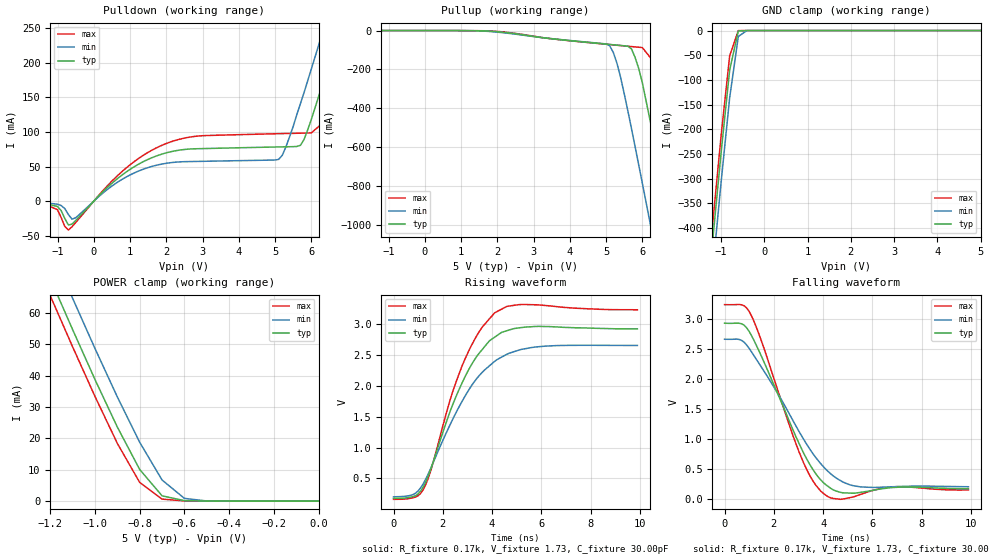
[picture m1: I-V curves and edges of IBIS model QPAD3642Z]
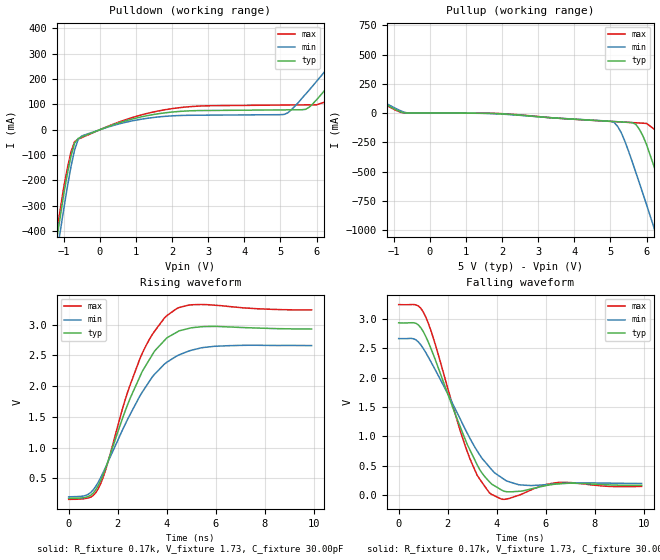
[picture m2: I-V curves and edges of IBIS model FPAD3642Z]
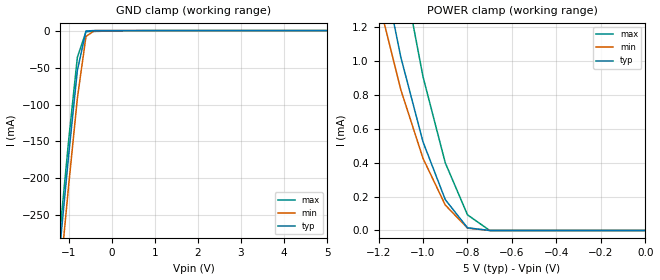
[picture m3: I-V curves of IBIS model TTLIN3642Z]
| IBIS file 723646.ibs created by s2ibis2 version 1.1
| North Carolina State University Electronics Research Laboratory  1995
[IBIS ver]   2.1
[File name]   723646.ibs
[File Rev]   1.0
[Date]   08/22/97
[Source]   Integrated Device Technology, Inc.
[Notes]   1. Temperatures: typ=25C, min=70C, max=0C 2. Cemos7_5v
   process. 3. Ramp rates based on 50 ohm load.
[Copyright]   Copyright 1997, Integrated Device Technology, Inc.
|   Component idt723646
[Component]   idt723646
[Manufacturer]   Integrated Device Technology
[Package]
| variable   typ   min   max
R_pkg   0.75   0.60   0.90
L_pkg   8.10nH   8.30nH   9.90nH
C_pkg   0.53pF   0.46pF   0.60pF
[Pin]  signal_name   model_name   R_pin   L_pin   C_pin
1   W_RA   TTLIN3642Z
2   ENA   TTLIN3642Z
3   CLKA   TTLIN3642Z
4   GND   GND
5   A35   QPAD3642Z
6   A34   QPAD3642Z
7   A33   QPAD3642Z
8   A32   QPAD3642Z
9   VCC   POWER
10   A31   QPAD3642Z
11   A30   QPAD3642Z
12   GND   GND
13   A29   QPAD3642Z
14   A28   QPAD3642Z
15   A27   QPAD3642Z
16   A26   QPAD3642Z
17   A25   QPAD3642Z
18   A24   QPAD3642Z
19   A23   QPAD3642Z
20   BEFWFTL   TTLIN3642Z
21   GND   GND
22   A22   QPAD3642Z
23   VCC   POWER
24   A21   QPAD3642Z
25   A20   QPAD3642Z
26   A19   QPAD3642Z
27   A18   QPAD3642Z
28   GND   GND
29   A17   QPAD3642Z
30   A16   QPAD3642Z
31   A15   QPAD3642Z
32   A14   QPAD3642Z
33   A13   QPAD3642Z
34   VCC   POWER
35   A12   QPAD3642Z
36   GND   GND
37   A11   QPAD3642Z
38   A10   QPAD3642Z
39   A9   QPAD3642Z
40   A8   QPAD3642Z
41   A7   QPAD3642Z
42   A6   QPAD3642Z
43   GND   GND
44   A5   QPAD3642Z
45   A4   QPAD3642Z
46   A3   QPAD3642Z
47   SPML   TTLIN3642Z
48   VCC   POWER
49   A2   QPAD3642Z
50   A1   QPAD3642Z
51   A0   QPAD3642Z
52   GND   GND
53   B0   QPAD3642Z
54   B1   QPAD3642Z
55   B2   QPAD3642Z
56   B3   QPAD3642Z
57   B4   QPAD3642Z
58   B5   QPAD3642Z
59   GND   GND
60   B6   QPAD3642Z
61   VCC   POWER
62   B7   QPAD3642Z
63   B8   QPAD3642Z
64   B9   QPAD3642Z
65   B10   QPAD3642Z
66   B11   QPAD3642Z
67   GND   GND
68   B12   QPAD3642Z
69   B13   QPAD3642Z
70   B14   QPAD3642Z
71   B15   QPAD3642Z
72   VCC   POWER
73   SIZEC   TTLIN3642Z
74   B16   QPAD3642Z
75   B17   QPAD3642Z
76   GND   GND
77   C0   QPAD3642Z
78   C1   QPAD3642Z
79   C2   QPAD3642Z
80   C3   QPAD3642Z
81   C4   QPAD3642Z
82   C5   QPAD3642Z
83   GND   GND
84   SIZEB   TTLIN3642Z
85   C6   QPAD3642Z
86   C7   QPAD3642Z
87   VCC   POWER
88   C8   QPAD3642Z
89   C9   QPAD3642Z
90   C10   QPAD3642Z
91   C11   QPAD3642Z
92   C12   QPAD3642Z
93   C13   QPAD3642Z
94   MBC   TTLIN3642Z
95   GND   GND
96   C14   QPAD3642Z
97   C15   QPAD3642Z
98   C16   QPAD3642Z
99   C17   QPAD3642Z
100   VCC   POWER
101   PRS2L   TTLIN3642Z
102   CLKB   TTLIN3642Z
103   ENB   TTLIN3642Z
104   W_RB   TTLIN3642Z
105   CSBL   TTLIN3642Z
106   GND   GND
107   FFCLIR   FPAD3642Z
108   EFBLOR   FPAD3642Z
109   AFCL   FPAD3642Z
110   AEBL   FPAD3642Z
111   VCC   POWER
112   MBF1   FPAD3642Z
113   MBB   TTLIN3642Z
114   MRS2L   TTLIN3642Z
115   FS1   TTLIN3642Z
116   GND   GND
117   CLKC   TTLIN3642Z
118   FS0   TTLIN3642Z
119   MRS1L   TTLIN3642Z
120   MBA   TTLIN3642Z
121   MBF2   FPAD3642Z
122   AEAL   FPAD3642Z
123   AFAL   FPAD3642Z
124   VCC   POWER
125   PRS1L   TTLIN3642Z
126   EFALOR   FPAD3642Z
127   FFALIR   FPAD3642Z
128   CSAL   TTLIN3642Z
| Models and submodels in the file (3): QPAD3642Z (I/O), FPAD3642Z (Output), TTLIN3642Z (Input)
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| FIN  FIN   dummy_model
| QIN  QIN   dummy_model
| QOEL QOEL   dummy_model
|   Model QPAD3642Z
[Model]   QPAD3642Z
Model_type   I/O
Polarity   Non-Inverting
Enable   Active-Low
Vinl =  0.000V
Vinh =  3.000V
Vmeas =  1.500V
C_comp   3.00pF   NA   NA
[Temperature Range]   25.00   70.00   0.000
[Voltage Range]   5.00V   4.50V   5.50V
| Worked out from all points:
|   slope of the pulldown table from 0 to 0.75 V, typ, clamps not added: 20.5 ohm
|   slope of the pullup table from 0 to 0.75 V, typ, clamps not added: 25.9 kohm
|   GND clamp passes 1 mA (typ) near -0.60 V on its own axis
|   POWER clamp passes 1 mA (typ) near -0.66 V on its own axis
|   rising waveform, R_fixture 0.17k, V_fixture 1.73, C_fixture 30.00pF: 20-80 % time 1.64ns typ, 1.93ns min, 1.5ns max; typ from 0.176 V to 2.93 V
|   falling waveform, R_fixture 0.17k, V_fixture 1.73, C_fixture 30.00pF: 20-80 % time 1.77ns typ, 2.16ns min, 1.53ns max; typ from 2.93 V to 0.173 V
[Pulldown]
| voltage   I(typ)   I(min)   I(max)
-5V       0A         -1mA       0A
-1.4V     -2.6mA     -1.9mA     -3.1mA
-1V       -7.7mA     -4.4mA     -12.4mA
-700mV    -34.39mA   -19.37mA   -41.73mA
700mV     34.57mA    28.94mA    39.05mA
1.8V      66.7mA     52.82mA    78.9mA
5.1V      78.42mA    60.43mA    97.58mA
5.7V      80.72mA    141mA      98.3mA
6.4V      184mA      259mA      117mA
6.8V      252mA      327mA      181mA
7.2V      320mA      396mA      249mA
10V       806mA      882mA      734mA
[Pullup]
| voltage   I(typ)   I(min)   I(max)
-5V       0A         0A         0A
1.8V      -3.202mA   -5.178mA   -2.04mA
5V        -69.89mA   -69.05mA   -70.44mA
5.1V      -71.61mA   -78.32mA   -72.17mA
5.3V      -75.05mA   -168mA     -75.61mA
5.7V      -94.45mA   -503mA     -82.44mA
6V        -268mA     -784mA     -87.54mA
6.4V      -630mA     -1.165A    -181mA
6.8V      -1.01A     -1.55A     -504mA
7.2V      -1.395A    -1.938A    -882mA
7.6V      -1.782A    -2.326A    -1.266A
10V       -4.125A    -4.67A     -3.606A
[GND_clamp]
| voltage   I(typ)   I(min)   I(max)
-5V       -4.123A    -4.179A    -4.092A
-1.4V     -620mA     -681mA     -587mA
-1.2V     -432mA     -493mA     -398mA
-1V       -249mA     -309mA     -215mA
-800mV    -80.04mA   -136mA     -51.24mA
-600mV    -972uA     -12mA      -154uA
-400mV    -331nA     -19.33uA   -23.45nA
5V        50nA       49.06uA    50nA
[POWER_clamp]
| voltage   I(typ)   I(min)   I(max)
-5V       723mA      732mA      718mA
-1.2V     70.9mA     80.87mA    65.4mA
-1.1V     54.63mA    64.6mA     49.14mA
-1V       38.73mA    48.62mA    33.34mA
-900mV    23.59mA    33.19mA    18.39mA
-800mV    10.08mA    18.74mA    5.951mA
-700mV    1.694mA    6.736mA    642uA
-600mV    151uA      876uA      70.05uA
-500mV    817nA      49.07uA    125nA
0V        50nA       45.12nA    55nA
[Ramp]
| variable   typ   min   max
dV/dt_r   1.07/0.80n   0.91/1.01n   1.23/0.70n
dV/dt_f   1.94/2.25n   1.56/2.83n   2.27/1.87n
R_load = 50.00
[Rising Waveform]
R_fixture = 0.17k
V_fixture = 1.73
C_fixture = 30.00pF
R_dut = 0.75
L_dut = 8.10nH
C_dut = 0.53pF
| time   V(typ)   V(min)   V(max)
0s        176mV      201mV      161mV
800ps     207mV      240mV      188mV
1.2ns     357mV      409mV      315mV
1.5ns     637mV      654mV      610mV
2.3ns     1.592V     1.374V     1.778V
2.8ns     2.064V     1.763V     2.343V
3.5ns     2.543V     2.179V     2.896V
4.1ns     2.791V     2.399V     3.185V
5.7ns     2.965V     2.63V      3.319V
9.9ns     2.928V     2.658V     3.237V
[Falling Waveform]
R_fixture = 0.17k
V_fixture = 1.73
C_fixture = 30.00pF
R_dut = 0.75
L_dut = 8.10nH
C_dut = 0.53pF
| time   V(typ)   V(min)   V(max)
0s        2.931V     2.664V     3.241V
600ps     2.93V      2.66V      3.243V
1ns       2.793V     2.511V     3.127V
1.5ns     2.377V     2.197V     2.632V
3.1ns     862mV      1.073V     710mV
4ns       280mV      546mV      98.93mV
4.7ns     114mV      310mV      -3.433mV
5.5ns     111mV      205mV      75.17mV
7ns       197mV      209mV      208mV
9.9ns     173mV      206mV      152mV
|   Model FPAD3642Z
[Model]   FPAD3642Z
Model_type   Output
Vmeas =  1.500V
C_comp   3.00pF   NA   NA
[Temperature Range]   25.00   70.00   0.000
[Voltage Range]   5.00V   4.50V   5.50V
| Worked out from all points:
|   slope of the pulldown table from 0 to 0.75 V, typ, clamps not added: 20.5 ohm
|   slope of the pullup table from 0 to 0.75 V, typ, clamps not added: 25.8 kohm
|   rising waveform, R_fixture 0.17k, V_fixture 1.73, C_fixture 30.00pF: 20-80 % time 1.65ns typ, 1.93ns min, 1.5ns max; typ from 0.176 V to 2.93 V
|   falling waveform, R_fixture 0.17k, V_fixture 1.73, C_fixture 30.00pF: 20-80 % time 1.54ns typ, 1.85ns min, 1.32ns max; typ from 2.93 V to 0.171 V
[Pulldown]
| voltage   I(typ)   I(min)   I(max)
-5V       -4.111A    -4.167A    -4.08A
-1.4V     -621mA     -681mA     -588mA
-1V       -255mA     -313mA     -227mA
-700mV    -53.07mA   -80.18mA   -47.24mA
-500mV    -28.01mA   -24.68mA   -30.93mA
1.9V      68.38mA    53.88mA    81.24mA
5.1V      78.42mA    60.43mA    97.58mA
5.7V      80.72mA    141mA      98.3mA
6.4V      184mA      259mA      117mA
7.6V      389mA      465mA      318mA
8.4V      528mA      604mA      456mA
10V       806mA      882mA      734mA
[Pullup]
| voltage   I(typ)   I(min)   I(max)
-5V       723mA      732mA      718mA
-800mV    10.08mA    18.74mA    5.951mA
1.9V      -4.537mA   -6.706mA   -3.085mA
5.1V      -71.61mA   -78.19mA   -72.17mA
5.3V      -75.05mA   -167mA     -75.61mA
5.7V      -94.3mA    -502mA     -82.44mA
6V        -268mA     -781mA     -87.54mA
6.4V      -628mA     -1.161A    -180mA
6.8V      -1.006A    -1.545A    -502mA
7.2V      -1.391A    -1.931A    -879mA
7.6V      -1.777A    -2.319A    -1.262A
10V       -4.112A    -4.655A    -3.595A
[Ramp]
| variable   typ   min   max
dV/dt_r   1.07/0.84n   0.91/1.03n   1.23/0.72n
dV/dt_f   1.96/1.74n   1.59/2.21n   2.28/1.43n
R_load = 50.00
[Rising Waveform]
R_fixture = 0.17k
V_fixture = 1.73
C_fixture = 30.00pF
R_dut = 0.75
L_dut = 8.10nH
C_dut = 0.53pF
| time   V(typ)   V(min)   V(max)
0s        176mV      201mV      161mV
800ps     206mV      244mV      184mV
1.2ns     380mV      435mV      330mV
1.5ns     661mV      677mV      631mV
2.4ns     1.697V     1.459V     1.899V
2.9ns     2.151V     1.838V     2.441V
3.5ns     2.569V     2.192V     2.891V
4ns       2.783V     2.387V     3.143V
5.5ns     2.967V     2.627V     3.324V
9.9ns     2.927V     2.658V     3.237V
[Falling Waveform]
R_fixture = 0.17k
V_fixture = 1.73
C_fixture = 30.00pF
R_dut = 0.75
L_dut = 8.10nH
C_dut = 0.53pF
| time   V(typ)   V(min)   V(max)
0s        2.931V     2.664V     3.241V
700ps     2.924V     2.643V     3.237V
1.1ns     2.703V     2.429V     3.034V
2.8ns     860mV      1.052V     737mV
3.2ns     517mV      754mV      341mV
3.7ns     228mV      480mV      40.98mV
4.2ns     88.14mV    299mV      -66.74mV
4.9ns     68mV       179mV      1.264mV
6.5ns     196mV      196mV      218mV
9.9ns     171mV      201mV      152mV
|   Model TTLIN3642Z
[Model]   TTLIN3642Z
Model_type   Input
Vinl =  0.000V
Vinh =  3.000V
Vmeas =  1.500V
C_comp   3.00pF   NA   NA
[Temperature Range]   25.00   70.00   0.000
[Voltage Range]   5.00V   4.50V   5.50V
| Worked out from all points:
|   GND clamp passes 1 mA (typ) near -0.60 V on its own axis
|   POWER clamp passes 1 mA (typ) near -1.10 V on its own axis
[GND_clamp]
| voltage   I(typ)   I(min)   I(max)
-5V       -2.772A    -2.809A    -2.759A
-1.2V     -290mA     -331mA     -270mA
-1V       -167mA     -208mA     -147mA
-800mV    -53.79mA   -91.48mA   -36.1mA
-600mV    -517uA     -7.891mA   -1.465mA
-400mV    -227nA     -13.17uA   -1.116mA
800mV     8nA        8.01nA     -40.1uA
5V        50nA       50.09nA    50nA
[POWER_clamp]
| voltage   I(typ)   I(min)   I(max)
-5V       69.72mA    59.04mA    81mA
-1.2V     1.67mA     1.357mA    2.454mA
-1.1V     1.022mA    830uA      1.596mA
-1V       522uA      425uA      906uA
-900mV    182uA      150uA      399uA
-800mV    15.59uA    13.98uA    92.07uA
-700mV    57nA       52.09nA    62nA
0V        50nA       45.08nA    55nA
